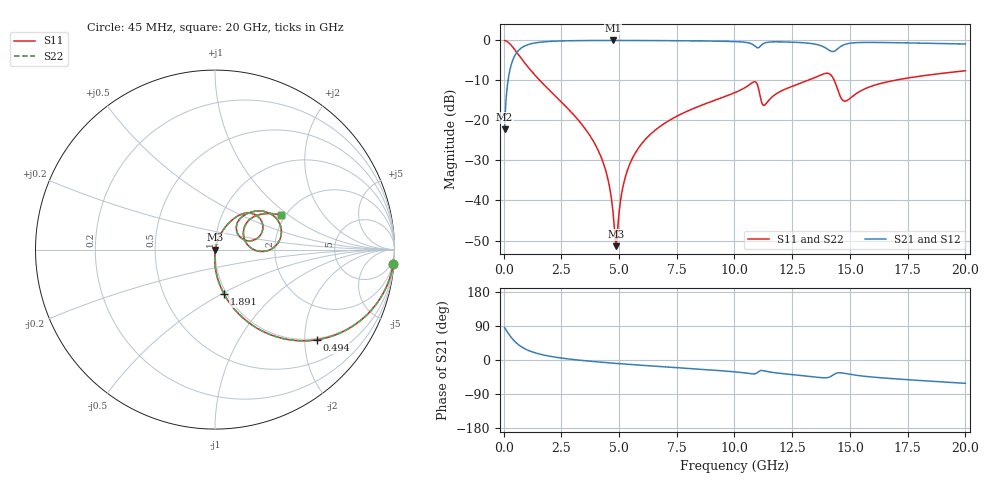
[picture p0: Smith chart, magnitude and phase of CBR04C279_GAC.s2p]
! S-parameter model data by Modelithics Inc.  support@modelithics.com 813-866-6335  Tampa FL USA
! S-Parameter data specifications:
! Substrate: 20-mil Rogers 4350B, substrate thickness, H=0.508mm, Dielectric constant, Er=3.75
! PCB Mounting Pad Footprint: Pad width, PadW=0.52mm , Pad length, PadL=0.52mm , Pad gap, PadG (edge-to-edge)=0.28mm , Reference planes=1.32mm apart
#  GHz  S  MA  R 50
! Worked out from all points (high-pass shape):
!   801 points, 45 MHz to 20 GHz, reference 50 ohm
!   highest |S21| = -0.02 dB at 4.734 GHz (marker M1); lowest = -22.2 dB at 45 MHz (marker M2)
!   |S21| within 3 dB of the highest: 574.6 MHz to end of sweep
!   lowest |S11| = -51.4 dB at 4.859 GHz (marker M3), VSWR 1.01, Z = 50.2 - j0.101 ohm
!   |S11| at or under -10 dB: 1.569 GHz to 13.18 GHz (11.61 GHz wide, 157 % of centre); 14.32 GHz to 16.92 GHz (2.6 GHz wide, 16.6 % of centre)
!   |S22| runs from -51.4 to 0.0 dB; largest |S21 - S12| = 0
!   S11 on the Smith chart (normalised r, x): 45 MHz: 1, -25; 494 MHz: 0.97, -2.29; 1.891 GHz: 0.97, -0.52; 20 GHz: 1.91, +0.88
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0.045  0.9969 -4.5  0.07721 85.4  0.07721 85.4  0.9969 -4.5
0.24455  0.921 -23.3  0.3876 66.6  0.3876 66.6  0.921 -23.3
0.493988  0.759 -41.4  0.6496 48.5  0.6496 48.5  0.759 -41.4
1.04275  0.4706 -63.7  0.8809 26.2  0.8809 26.2  0.4706 -63.7
1.890837  0.2538 -78.4  0.9655 11.2  0.9655 11.2  0.2538 -78.4
3.387462  0.08935 -89.7  0.9937 -1.1  0.9937 -1.1  0.08935 -89.7
4.310381  0.02991 -91.5  0.997 -6.2  0.997 -6.2  0.02991 -91.5
4.559819  0.01631 -88.5  0.9972 -7.5  0.9972 -7.5  0.01631 -88.5
4.734425  0.00742 -78.0  0.9972 -8.3  0.9972 -8.3  0.00742 -78.0
4.859144  0.002687 -22.0  0.9972 -8.9  0.9972 -8.9  0.002687 -22.0
4.933975  0.004093 40.6  0.9972 -9.3  0.9972 -9.3  0.004093 40.6
5.158469  0.01431 68.8  0.997 -10.3  0.997 -10.3  0.01431 68.8
5.457794  0.02816 72.7  0.9966 -11.6  0.9966 -11.6  0.02816 72.7
6.704981  0.08121 70.8  0.9933 -17.0  0.9933 -17.0  0.08121 70.8
10.0225  0.2229 56.3  0.9653 -31.3  0.9653 -31.3  0.2229 56.3
10.87059  0.3043 33.8  0.8559 -36.6  0.8559 -36.6  0.3043 33.8
11.29463  0.1547 35.7  0.9231 -28.8  0.9231 -28.8  0.1547 35.7
13.36496  0.3324 40.3  0.9097 -43.9  0.9097 -43.9  0.3324 40.3
14.11327  0.3813 14.1  0.7487 -45.0  0.7487 -45.0  0.3813 14.1
14.78676  0.1739 20.1  0.8907 -35.4  0.8907 -35.4  0.1739 20.1
16.68248  0.3061 38.9  0.9378 -48.5  0.9378 -48.5  0.3061 38.9
20  0.4169 27.3  0.9 -61.5  0.9 -61.5  0.4169 27.3
